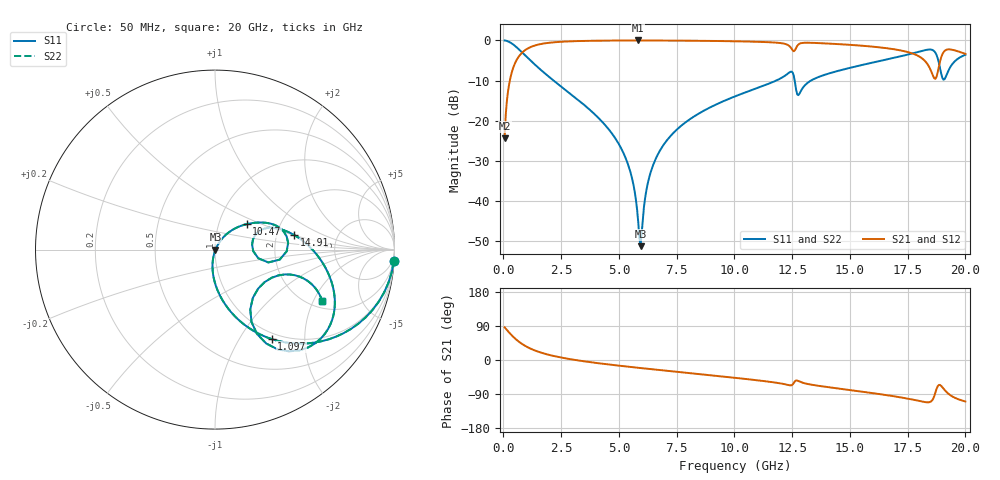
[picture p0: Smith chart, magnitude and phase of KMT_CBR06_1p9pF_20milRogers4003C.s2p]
! Data measured by Modelithics Inc. support@modelithics.com 813-866-6335
! KEMET CBR0603 1.9pF, Pad Width= 0.851mm, Pad Length= 0.64mm, Pad Gap= 0.62mm, 20mil Rogers 4003C substrate Data, January 2022
# hz S ma R 50
! 2 Port Network Data from SP1.SP block
! freq  magS11  angS11  magS21  angS21  magS12  angS12  magS22  angS22
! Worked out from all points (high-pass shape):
!   401 points, 50 MHz to 20 GHz, reference 50 ohm
!   highest |S21| = -0.03 dB at 5.835 GHz (marker M1); lowest = -24.4 dB at 50 MHz (marker M2)
!   |S21| within 3 dB of the highest: 812.5 MHz to 17.58 GHz (16.77 GHz wide, 182 % of centre); 19.04 GHz to 19.84 GHz (795.6 MHz wide, 4.09 % of centre)
!   lowest |S11| = -51.2 dB at 5.935 GHz (marker M3), VSWR 1.01, Z = 50.3 - j0.0595 ohm
!   |S11| at or under -10 dB: 2.173 GHz to 11.8 GHz (9.631 GHz wide, 138 % of centre); 12.61 GHz to 13.31 GHz (702.6 MHz wide, 5.42 % of centre)
!   |S22| runs from -51.2 to 0.0 dB; largest |S21 - S12| = 0
!   S11 on the Smith chart (normalised r, x): 50 MHz: 1, -31; 1.097 GHz: 0.91, -1.39; 10.47 GHz: 1.36, +0.41; 14.91 GHz: 2.51, +0.51; 20 GHz: 2.30, -2.35
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5e7  0.9982 -3.6  0.06034 86.3  0.06034 86.3  0.9982 -3.6
3.99125e8  0.8996 -27.3  0.4358 62.7  0.4358 62.7  0.8996 -27.3
1.097375e9  0.5892 -57.7  0.8065 32.2  0.8065 32.2  0.5892 -57.7
3.391625e9  0.1668 -91.8  0.9837 -2.6  0.9837 -2.6  0.1668 -91.8
5.187125e9  0.04027 -102.6  0.9964 -16.2  0.9964 -16.2  0.04027 -102.6
5.586125e9  0.01824 -100.5  0.997 -18.9  0.997 -18.9  0.01824 -100.5
5.8355e9  0.005492 -81.0  0.9971 -20.5  0.9971 -20.5  0.005492 -81.0
5.93525e9  0.002761 -12.4  0.9971 -21.2  0.9971 -21.2  0.002761 -12.4
6.284375e9  0.01846 57.8  0.9968 -23.4  0.9968 -23.4  0.01846 57.8
6.73325e9  0.04058 59.6  0.996 -26.3  0.996 -26.3  0.04058 59.6
1.0025e10  0.2013 41.8  0.9751 -47.0  0.9751 -47.0  0.2013 41.8
1.047388e10  0.2256 38.9  0.9694 -50.0  0.9694 -50.0  0.2256 38.9
1.2419e10  0.4058 10.4  0.8283 -66.8  0.8283 -66.8  0.4058 10.4
1.26185e10  0.3056 -13.5  0.753 -56.1  0.753 -56.1  0.3056 -13.5
1.336662e10  0.3228 22.1  0.9324 -65.5  0.9324 -65.5  0.3228 22.1
1.491275e10  0.449 10.4  0.8842 -78.5  0.8842 -78.5  0.449 10.4
1.670825e10  0.5896 -5.3  0.7913 -93.8  0.7913 -93.8  0.5896 -5.3
1.830425e10  0.7617 -31.2  0.5318 -111.5  0.5318 -111.5  0.7617 -31.2
1.870325e10  0.7009 -54.0  0.3329 -85.7  0.3329 -85.7  0.7009 -54.0
1.895262e10  0.3864 -59.4  0.6158 -68.3  0.6158 -68.3  0.3864 -59.4
1.925188e10  0.4121 -19.6  0.7736 -88.4  0.7736 -88.4  0.4121 -19.6
2e10  0.663 -25.6  0.6802 -109.5  0.6802 -109.5  0.663 -25.6
